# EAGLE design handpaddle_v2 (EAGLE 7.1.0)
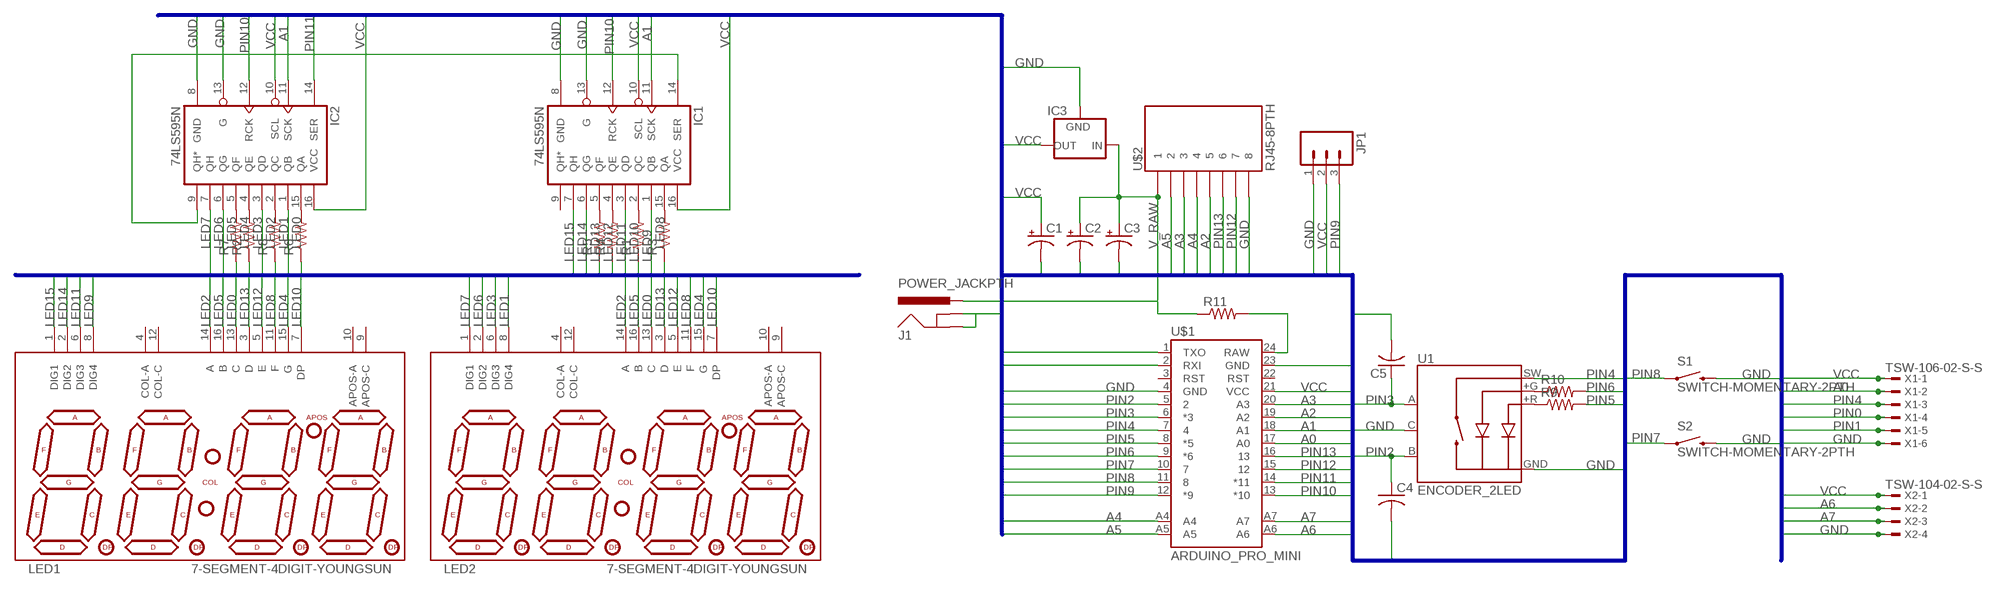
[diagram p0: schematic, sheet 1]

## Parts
C1  CPOL-USE2.5-6  [E2,5-6]
C2  CPOL-USE2.5-6  [E2,5-6]
C3  CPOL-USE2.5-6  [E2,5-6]
C4  C-USC0805  [C0805]
C5  C-USC0805  [C0805]
IC1  74LS595N  [DIL16]
IC2  74LS595N  [DIL16]
IC3  V_REG_78XXSINK  [TO220-IGO]
J1  POWER_JACKPTH  [POWER_JACK_PTH]
JP1  M03PTH  [1X03]
LED1  7-SEGMENT-4DIGIT-YOUNGSUN  [7-SEGMENT-4DIGIT-YOUNGSUN]
LED2  7-SEGMENT-4DIGIT-YOUNGSUN  [7-SEGMENT-4DIGIT-YOUNGSUN]
R1  R-US_R0805  [R0805]
R2  R-US_R0805  [R0805]
R3  R-US_R0805  [R0805]
R4  R-US_R0805  [R0805]
R5  R-US_R0805  [R0805]
R6  R-US_R0805  [R0805]
R7  R-US_R0805  [R0805]
R8  R-US_R0805  [R0805]
R9  R-US_R0805  [R0805]
R10  R-US_R0805  [R0805]
R11  R-US_R0805  [R0805]
S1  SWITCH-MOMENTARY-2PTH  [TACTILE-PTH]
S2  SWITCH-MOMENTARY-2PTH  [TACTILE-PTH]
U1  ENCODER_2LED  [ENCODER_LED_2]
U$1  ARDUINO_PRO_MINI  [ARDUINO_PRO_MINI]
U$2  RJ45-8PTH  [RJ45-8]
X1  TSW-106-02-S-S  [TSW-106-02-S-S]
X2  TSW-104-02-S-S  [TSW-104-02-S-S]

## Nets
A0: U$1.17(A0) X1.2
A1: IC1.11(SCK) IC2.11(SCK) U$1.18(A1)
A2: U$1.19(A2) U$2.5
A3: U$1.20(A3) U$2.3
A4: U$1.A4 U$2.4
A5: U$1.A5 U$2.2
A6: U$1.A6 X2.2
A7: U$1.A7 X2.3
GND: C1.- C2.- C3.- C4.2 C5.2 IC1.8(GND) IC1.13(G) IC2.8(GND) IC2.13(G) IC3.GND J1.GND J1.GNDBREAK JP1.1 S1.3 S2.3 U1.C U1.GND(-) U$1.4(GND) U$1.23(GND) U$2.8 X1.6 X2.4
LED0: LED1.13(C) LED2.13(C) R6.1
LED1: IC2.1(QB) LED2.8(DIG4)
LED2: LED1.14(A) LED2.14(A) R8.1
LED3: IC2.3(QD) LED2.6(DIG3)
LED4: LED1.15(G) LED2.15(G) R2.1
LED5: LED1.16(B) LED2.16(B) R7.1
LED6: IC2.6(QG) LED2.2(DIG2)
LED7: IC2.7(QH) LED2.1(DIG1)
LED8: LED1.11(F) LED2.11(F) R3.1
LED9: IC1.1(QB) LED1.8(DIG4)
LED10: LED1.7(DP) LED2.7(DP) R1.1
LED11: IC1.3(QD) LED1.6(DIG3)
LED12: LED1.5(E) LED2.5(E) R4.1
LED13: LED1.3(D) LED2.3(D) R5.1
LED14: IC1.6(QG) LED1.2(DIG2)
LED15: IC1.7(QH) LED1.1(DIG1)
N$1: IC1.14(SER) IC2.9(QH*)
N$2: IC2.5(QF) R7.2
N$3: IC2.4(QE) R2.2
N$4: IC2.2(QC) R8.2
N$5: IC2.15(QA) R6.2
N$6: IC1.15(QA) R3.2
N$7: IC1.2(QC) R1.2
N$8: IC1.4(QE) R4.2
N$9: IC1.5(QF) R5.2
N$10: R11.2 U$1.24(RAW)
N$11: R9.1 U1.+R
N$12: R10.1 U1.+G
PIN0: U$1.1(TXO) X1.4
PIN1: U$1.2(RXI) X1.5
PIN2: C4.1 U1.B U$1.5
PIN3: C5.1 U1.A U$1.6(*3)
PIN4: U1.SW U$1.7 X1.3
PIN5: R9.2 U$1.8(*5)
PIN6: R10.2 U$1.9(*6)
PIN7: S2.1 U$1.10
PIN8: S1.1 U$1.11
PIN9: JP1.3 U$1.12(*9)
PIN10: IC1.12(RCK) IC2.12(RCK) U$1.13(*10)
PIN11: IC2.14(SER) U$1.14(*11)
PIN12: U$1.15 U$2.7
PIN13: U$1.16 U$2.6
V_RAW: C2.+ C3.+ IC3.IN J1.PWR R11.1 U$2.1
VCC: C1.+ IC1.10(SCL) IC1.16(VCC) IC2.10(SCL) IC2.16(VCC) IC3.OUT JP1.2 U$1.21(VCC) X1.1 X2.1
Unconnected: IC1.9(QH*) LED1.4(COL-A) LED1.9(APOS-C) LED1.10(APOS-A) LED1.12(COL-C) LED2.4(COL-A) LED2.9(APOS-C) LED2.10(APOS-A) LED2.12(COL-C) U$1.3(RST) U$1.22(RST)

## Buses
LED[0..15]
PIN[0..13],A[0..7],VCC,GND

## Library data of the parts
C1-C3 = rcl:CPOL-US: POLARIZED CAPACITOR, American symbol
C4 C5 = rcl:C-US: CAPACITOR, American symbol
IC1 IC2 = SparkFun-DigitalIC:74*595: 8-bit SHIFT REGISTER, output latch
IC3 = SparkFun-PowerIC:V_REG_78XX: Voltage Regulator Standard 7805 5V regulator. IGO (Input Ground Output). Spark Fun Electronics SKU : COM-00107
J1 = SparkFun-Connectors:POWER_JACK: Power Jack This is the standard 5.5mm barrel jack for power. The PTH is the most common, proven, reliable, footprint. The Slot footprint only works if the mill layer is transmitted to the PCB fab house so be warned. Mating wall wart : TOL-00298 (and others); PROD_ID: PRT-00119
JP1 = SparkFun-Connectors:M03: Header 3 Standard 3-pin 0.1" header. Use with straight break away headers (SKU : PRT-00116), right angle break away headers (PRT-00553), swiss pins (PRT-00743), machine pins (PRT-00117), and female headers (PRT-00115). Molex polarized connector foot print use with SKU : PRT-08232 with associated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
LED1 LED2 = SparkFun-Displays:7-SEGMENT-4DIGIT-YOUNGSUN: This is a part for the 4-Digit 7-segment LEDs from Young Sun. Different from the Digikey LEDs, all 16 pins are used. The LONGPADS Variant is used for a test jig, but you may like it because there is more pad to solder to. If you are concerned about routing space, the standard works just fine though.
R1-R11 = rcl:R-US_: RESISTOR, American symbol
S1 S2 = SparkFun-Electromechanical:SWITCH-MOMENTARY-2: Various NO switches- pushbuttons, reed, etc
U1 = SparkFun-Electromechanical:ENCODER_2LED: Illuminated Rotary Encoder w/ 2 LEDs
U$1 = SparkFun-Boards:ARDUINO_PRO_MINI
U$2 = SparkFun-Connectors:RJ45-8: RJ45 Jack Simple RJ45, 8-pin connection - connector for common Cat5, Cat5e, and Cat6 Ethernet cables. Footprint not yet proven in production. Connector sku is PRT-00643; Breakout PCB sku is BOB-00716.
X1 = con-samtec:TSW-106-02-S-S: THROUGH-HOLE .025" SQ POST HEADER Source: Samtec TSW.pdf; OC_FARNELL: unknown; OC_NEWARK: unknown
X2 = con-samtec:TSW-104-02-S-S: THROUGH-HOLE .025" SQ POST HEADER Source: Samtec TSW.pdf; OC_FARNELL: unknown; OC_NEWARK: unknown

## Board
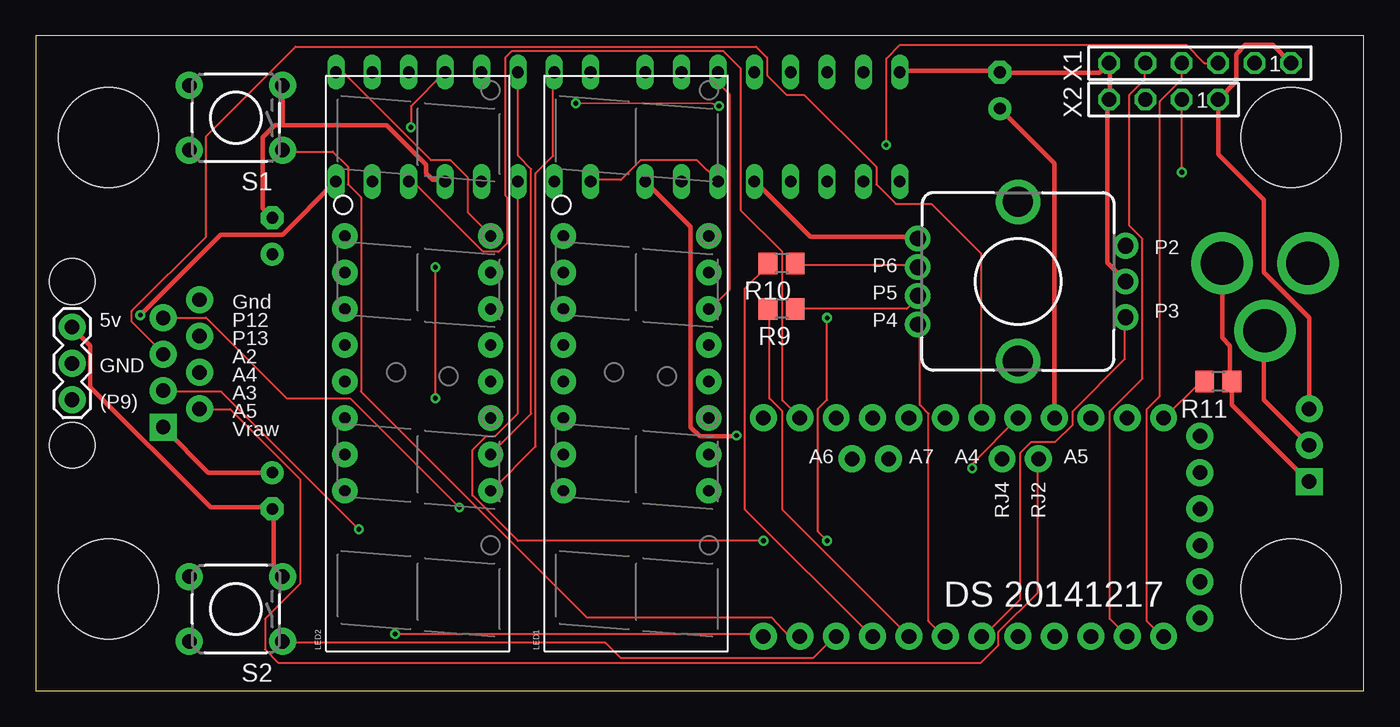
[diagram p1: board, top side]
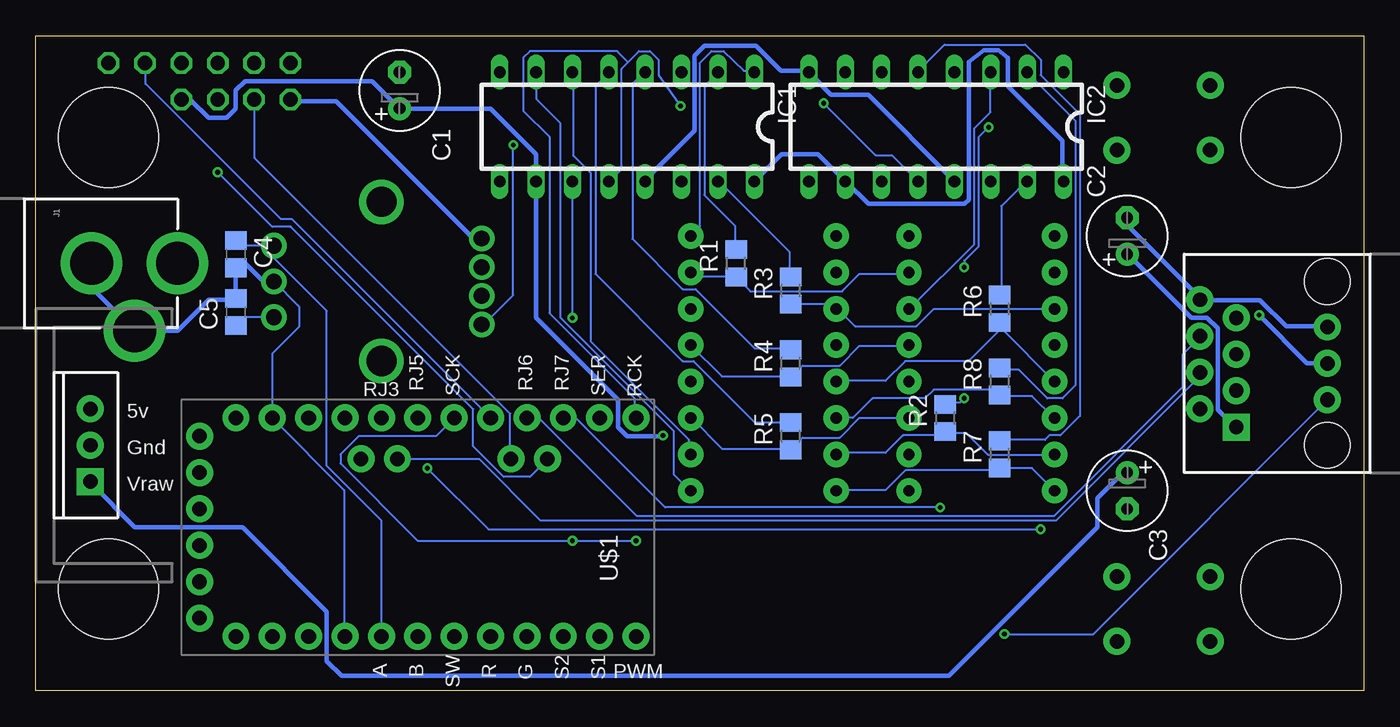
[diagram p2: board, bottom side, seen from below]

Size 92.71 x 45.72 mm. Coordinates in mm from the lower left corner, seen from the top.
Outline: 0,0 92.71,0 92.71,45.72 0,45.72 0,0
Copper layers (1*16): Top 0.0356mm / dielectric 1.5011mm / Bottom 0.0356mm
Design rules "LaenPCBOrder": minimum track width 6mil, minimum drill 13mil, track to track 6mil, track to pad 6mil, pad to pad 6mil, via to via 6mil, smd to smd 6mil, copper to edge 15mil, drill to drill 6mil, minimum pad ring 7mil, minimum via ring 7mil, stop-mask expansion 3mil, vias tented up to drill 0mil, thermal gap 10mil
Holes 6.99 mm at 5.08,38.61 5.08,7.11 87.63,38.61 87.63,7.11

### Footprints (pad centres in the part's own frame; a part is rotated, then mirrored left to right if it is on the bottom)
E2,5-6 = drill 0.813 pad 1.6: + -1.27,0 | drill 0.813 pad 1.6 octagon: - 1.27,0
C0805 = smd 1.3 x 1.5: 1 -0.95,0; 2 0.95,0
DIL16 = drill 0.813 long: 1 -8.89,-3.81; 2 -6.35,-3.81; 3 -3.81,-3.81; 4 -1.27,-3.81; 5 1.27,-3.81; 6 3.81,-3.81; 7 6.35,-3.81; 8 8.89,-3.81; 9 8.89,3.81; 10 6.35,3.81; 11 3.81,3.81; 12 1.27,3.81; 13 -1.27,3.81; 14 -3.81,3.81; 15 -6.35,3.81; 16 -8.89,3.81
TO220-IGO = drill 1 pad 1.88: GND 0,0; OUT 2.54,0 | drill 1 pad 1.88 square: IN -2.54,0
POWER_JACK_PTH = drill 2.997 pad 4.318: GND 0,7.7; GNDBREAK 4.7,10.7; PWR 0,13.7
1X03 = drill 1.016 pad 1.88: 1 0,0; 2 2.54,0; 3 5.08,0
7-SEGMENT-4DIGIT-YOUNGSUN = drill 0.8 pad 1.778: 1 -8.89,-5.08; 2 -6.35,-5.08; 3 -3.81,-5.08; 4 -1.27,-5.08; 5 1.27,-5.08; 6 3.81,-5.08; 7 6.35,-5.08; 8 8.89,-5.08; 9 8.89,5.08; 10 6.35,5.08; 11 3.81,5.08; 12 1.27,5.08; 13 -1.27,5.08; 14 -3.81,5.08; 15 -6.35,5.08; 16 -8.89,5.08
R0805 = smd 1.3 x 1.5: 1 -0.95,0; 2 0.95,0
TACTILE-PTH = drill 1.016 pad 1.88: 1 -3.251,2.261; 2 3.251,2.261; 3 -3.251,-2.261; 4 3.251,-2.261
ENCODER_LED_2 = drill 1.1 pad 1.778: +G 1,7; +R -1,7; GND 3,7; SW -3,7 | drill 1.1 pad 1.8: A -2.5,-7.5; B 2.5,-7.5; C 0,-7.5 | drill 2.1: P$1 -5.55,0; P$2 5.55,0
ARDUINO_PRO_MINI = drill 1.016 pad 1.88: 1 -7.62,12.7; 2 -7.62,10.16; 3 -7.62,7.62; 4 -7.62,5.08; 5 -7.62,2.54; 6 -7.62,0; 7 -7.62,-2.54; 8 -7.62,-5.08; 9 -7.62,-7.62; 10 -7.62,-10.16; 11 -7.62,-12.7; 12 -7.62,-15.24; 13 7.62,-15.24; 14 7.62,-12.7; 15 7.62,-10.16; 16 7.62,-7.62; 17 7.62,-5.08; 18 7.62,-2.54; 19 7.62,0; 20 7.62,2.54; 21 7.62,5.08; 22 7.62,7.62; 23 7.62,10.16; 24 7.62,12.7; A4 4.763,1.429; A5 4.763,3.969; A6 4.763,-9.049; A7 4.763,-6.509; BLK -6.35,15.24; GND -3.81,15.24; GRN 6.35,15.24; RXI 1.27,15.24; TXO 3.81,15.24; VCC -1.27,15.24
RJ45-8 = drill 1 pad 1.88 square: 1 -4.445,6.35 | drill 1 pad 1.88: 2 -3.175,8.89; 3 -1.905,6.35; 4 -0.635,8.89; 5 0.635,6.35; 6 1.905,8.89; 7 3.175,6.35; 8 4.445,8.89 | hole 3.2: -5.715,0; 5.715,0
TSW-106-02-S-S = drill 1 pad 1.5 octagon: 1 6.35,0; 2 3.81,0; 3 1.27,0; 4 -1.27,0; 5 -3.81,0; 6 -6.35,0
TSW-104-02-S-S = drill 1 pad 1.5 octagon: 1 3.81,0; 2 1.27,0; 3 -1.27,0; 4 -3.81,0

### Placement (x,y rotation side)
C1  67.31,41.91 90 bottom
C2  16.51,31.75 90 bottom
C3  16.51,13.97 270 bottom
C4  78.74,30.48 270 bottom
C5  78.74,26.44 90 bottom
IC1  51.44,39.37 180 bottom
IC2  29.84,39.37 180 bottom
IC3  88.9,17.14 90 bottom
J1  96.52,29.84 270 bottom
JP1  2.54,25.4 270 top
LED1  41.91,22.86 90 top
LED2  26.67,22.86 90 top
R1  43.81,29.84 90 bottom
R2  29.21,19.05 90 bottom
R3  40.01,27.94 90 bottom
R4  40.01,22.86 90 bottom
R5  40.01,17.78 90 bottom
R6  25.4,26.67 90 bottom
R7  25.4,16.51 90 bottom
R8  25.4,21.59 90 bottom
R9  52.07,26.67 180 top
R10  52.07,29.84 180 top
R11  82.55,21.59 180 top
S1  13.97,40.01 180 top
S2  13.97,5.71 180 top
U1  68.58,28.57 90 top
U$1  66.04,11.43 90 bottom
U$2  2.54,22.86 90 bottom
X1  81.28,43.81 0 top
X2  78.74,41.27 0 top

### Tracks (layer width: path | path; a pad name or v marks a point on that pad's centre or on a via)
A0
  Bottom 0.152: U$1.17 74.83,32.92 75.59,32.92 85.04,42.37 85.04,43.74 X1.2
A1  (via drill 0.33)
  Top 0.152: IC2.11 33.66,19.37 32.07,17.78 31.43,17.78 30.48,16.83 30.48,13.65 33.66,10.48 v50.8,10.48 | v55.24,26.04 55.24,20.32 54.61,19.68 54.61,11.11 v55.24,10.48
  Bottom 0.152: v50.8,10.48 v55.24,10.48 66.04,10.48 71.44,15.88 71.44,16.51 70.17,17.78 64.77,17.78 U$1.18 | v55.24,26.04 IC1.11
A2
  Top 0.152: U$1.19 65.99,19.05 65.99,30.53 62.53,33.98 60.05,33.98 58.67,35.36 58.67,36.58 53.65,41.6 52.43,41.6 51.05,42.98 51.05,44.2 50.29,44.96 18.14,44.96 11.89,38.71 11.89,31.7 6.71,26.52 6.71,25.76 8.84,23.62 U$2.5
A3  (via drill 0.33)
  Top 0.152: v22.55,11.28 12.95,20.88 8.99,20.88 U$2.3 | v65.38,15.54 65.38,15.85 U$1.20
  Bottom 0.152: v22.55,11.28 61.11,11.28 v65.38,15.54
A4
  Bottom 0.152: U$2.4 11.43,21.95 21.49,11.89 57.45,11.89 61.72,16.15 67.36,16.15 U$1.A4
A5
  Top 0.152: U$1.A5 69.95,16.15 69.95,6.86 67.21,4.12 67.21,3.2 65.99,1.98 16.92,1.98 16,2.9 16,5.03 18.44,7.47 18.44,14.78 13.56,19.66 11.43,19.66 U$2.2
A6  (via drill 0.33)
  Top 0.152: v80.01,36.2 X2.2
  Bottom 0.152: 80.01,41.3 X2.2 | U$1.A6 57,16.15 58.22,14.94 60.05,14.94 62.18,17.07 62.18,19.66 74.92,32.4 74.93,32.38 76.2,32.38 v80.01,36.2
A7
  Bottom 0.152: X2.3 77.42,41.15 77.42,37.19 59.59,19.36 59.59,16.31 U$1.A7
GND
  Top 0.152: 16.61,12.65 C3.- 16.46,12.8 | 17.22,8.08 S2.3 | 2.59,25.3 JP1.1 | 28.5,35.66 IC2.13 | 50.29,35.51 IC1.13 | 61.57,31.7 U1.GND | 74.98,41.3 X2.4 74.83,41.15 | 60.35,43.28 IC1.8 | 67.21,43.28 C1.- 67.36,43.13 | 76.05,28.65 U1.C | 74.98,43.74 74.98,43.13 X1.6 74.98,43.74
  Top 0.305: 16.61,12.65 16.61,8.69 17.22,8.08 | 17.22,39.47 S1.3 | C2.- 15.85,33.68 15.85,38.65 16.67,39.47 17.22,39.47 | 16.46,12.8 12.19,12.8 3.81,21.18 3.81,24.08 2.59,25.3 | 28.5,35.66 27.71,35.66 27.25,36.12 27.25,36.62 27.23,36.64 27.23,36.73 24.49,39.47 17.22,39.47 | 50.29,35.51 54.1,31.7 61.57,31.7 | 67.21,43.28 60.35,43.28 | 74.83,41.15 74.83,29.87 76.05,28.65 | IC3.GND 85.72,20.32 85.72,25.05 J1.GNDBREAK | 67.36,43.13 74.24,43.13 X1.6 | 74.98,43.13 74.98,41.33 X2.4
  Bottom 0.152: 38.71,43.13 IC2.8 38.86,43.28 | 16.46,32.92 C2.- | 11.43,27.43 U$2.8 11.43,27.28 | 2.59,25.45 JP1.1 | 61.72,31.7 U1.GND | 74.83,41.15 X2.4 | U$1.4 71.17,3.81 71.17,14.02 U$1.23 76.2,23.55 74.3,25.45 74.3,26.79 74.39,26.88 U1.C | 50.14,35.66 IC1.13
  Bottom 0.305: 38.71,43.13 37.19,41.6 34.58,41.6 28.67,35.68 28.65,35.66 IC2.13 | 16.46,32.92 16.46,32.46 11.43,27.43 | 2.59,25.45 5.41,25.45 7.24,27.28 11.43,27.28 | 61.72,31.7 62.28,31.7 71.73,41.15 74.83,41.15 | 38.86,43.28 40.68,43.28 42.43,45.03 46.01,45.03 46.71,44.33 46.71,39.09 50.14,35.66 | U1.C 76.83,28.57 78.11,29.84 78.42,29.84 C4.2 C5.2 78.83,27.3 80.64,27.3 82.81,25.14 J1.GNDBREAK 88.82,28.14 J1.GND
LED0
  Bottom 0.152: 25.3,25.3 25.3,25.6 R6.1 25.3,25.3 | LED2.13 25.3,25.3 | 25.3,25.3 27.58,23.01 32,23.01 33.38,21.64 36.73,21.64 LED1.13
LED1
  Top 0.152: IC2.1 21.03,43.13 21.49,43.13 27.58,37.03 28.96,37.03 30.18,35.81 30.18,33.38 31.7,31.85 LED2.8
LED2
  Bottom 0.152: LED2.14 21.64,19.05 23.16,20.57 25.3,20.57 R8.1 25.45,20.73 25.76,21.03 30.02,21.03 30.63,20.42 34.29,20.42 35.66,19.05 LED1.14
LED3
  Bottom 0.152: IC2.3 26.06,43.13 26.06,40.39 27.19,39.25 27.19,31.18 31.7,26.67 LED2.6
LED4
  Bottom 0.152: LED2.15 21.64,16.46 26.21,16.46 27.74,17.98 29.11,17.98 R2.1 29.26,17.98 29.41,17.83 32.16,17.83 33.38,16.61 36.73,16.61 LED1.15
LED5
  Bottom 0.152: LED2.16 23.16,15.54 25.3,15.54 R7.1 25.45,15.54 25.6,15.39 32,15.39 33.38,14.02 36.73,14.02 LED1.16
LED6
  Top 0.152: LED2.2 34.59,19.36 34.59,36.42 33.68,37.34 33.68,43.13 IC2.6
LED7
  Top 0.152: IC2.7 36.12,43.13 36.12,37.34 34.9,36.12 34.9,17.07 31.85,14.02 LED2.1
LED8
  Bottom 0.152: R3.1 39.93,26.98 37.19,26.98 36.88,26.67 LED1.11 36.73,26.67 35.51,25.45 31.24,25.45 30.02,26.67 LED2.11
LED9
  Bottom 0.152: IC1.1 42.67,43.28 43.28,43.28 44.68,44.65 45.54,44.65 46.33,43.84 46.33,32.46 46.94,31.85 LED1.8
LED10
  Bottom 0.152: LED1.7 46.94,29.11 46.79,28.96 43.89,28.96 R1.1 43.74,28.8 42.82,27.89 36.42,27.89 35.2,29.11 31.85,29.11 LED2.7
LED11
  Top 0.152: IC1.3 47.7,43.13 47.7,42.37 48.46,41.6 48.46,28.04 47.09,26.67 LED1.6
LED12
  Bottom 0.152: LED1.5 44.81,21.95 40.08,21.95 R4.1 39.93,21.95 39.17,22.71 36.58,22.71 35.2,24.08 31.85,24.08 LED2.5
LED13
  Bottom 0.152: LED1.3 46.94,19.05 44.81,16.92 40.08,16.92 R5.1 39.93,16.92 39.17,17.68 36.58,17.68 35.2,19.05 LED2.3
LED14
  Bottom 0.152: IC1.6 55.17,43.13 55.17,37.34 53.95,36.12 53.95,24.38 47.09,17.53 47.09,16.61 LED1.2
LED15
  Bottom 0.152: IC1.7 57.76,43.13 57.76,41.3 56.08,39.62 56.08,26.06 48.16,18.14 48.16,15.09 47.09,14.02 LED1.1
N$1
  Top 0.152: IC2.9 38.86,35.66 40.84,35.66 42.22,37.03 46.18,37.03 47.55,35.66 IC1.14
N$2
  Bottom 0.152: R7.2 25.3,17.53 22.25,17.53 21.95,17.83 21.18,17.83 19.81,19.2 19.81,40.23 22.55,42.98 22.55,44.04 23.62,45.11 29.26,45.11 31.09,43.28 IC2.5
N$3  (via drill 0.33)
  Top 0.152: v27.89,29.57 v27.89,20.42 | v26.19,39.34 26.19,40.82 28.5,43.13 IC2.4
  Bottom 0.152: v27.89,20.42 28.19,20.12 29.11,20.12 R2.2 | v27.89,29.57 27.89,30.02 26.89,31.01 26.89,38.64 v26.19,39.34
N$4
  Bottom 0.152: R8.2 25.3,22.4 24.08,22.4 22.1,20.42 21.03,20.42 20.12,21.34 20.12,39.78 23.47,43.13 IC2.2
N$5
  Bottom 0.152: R6.2 25.3,27.74 25.3,33.83 23.62,35.51 IC2.15
N$6
  Bottom 0.152: R3.2 40.08,28.96 40.08,30.63 44.96,35.51 IC1.15
N$7
  Bottom 0.152: R1.2 43.89,30.94 43.89,32.46 46.02,34.59 46.02,42.22 45.11,43.13 IC1.2
N$8
  Bottom 0.152: R4.2 40.08,23.93 42.52,23.93 46.63,28.04 47.55,28.04 51.05,31.55 51.05,42.37 50.29,43.13 IC1.4
N$9
  Bottom 0.152: R5.2 40.08,18.75 42.52,18.75 46.79,23.01 47.55,23.01 53.65,29.11 53.65,42.22 52.73,43.13 IC1.5
N$10
  Top 0.152: R11.2 81.53,21.49 81.23,21.49 78.79,19.05 U$1.24
N$11
  Top 0.152: R9.1 60.81,26.67 61.57,27.43 U1.+R
N$12
  Top 0.152: R10.1 53.03,29.72 61.57,29.72 U1.+G
PIN0
  Top 0.152: X1.4 80.01,42.67 78.49,41.15 78.49,20.57 77.57,19.66 77.57,4.88 78.64,3.81 U$1.1
PIN1
  Top 0.152: U$1.2 74.98,5.03 74.98,19.51 77.27,21.79 77.27,31.55 76.35,32.46 76.35,41.6 77.42,42.67 77.42,43.74 X1.5
PIN2
  Bottom 0.152: U$1.5 68.58,11.89 72.39,15.7 72.39,26.52 76.05,30.18 76.05,30.94 U1.B 78.39,31.07 C4.1
PIN3
  Top 0.152: U1.A 76.05,26.06 76.05,23.16 72.39,19.51 72.39,18.59 71.17,17.37 69.49,17.37 68.73,16.61 68.73,6.4 66.14,3.81 U$1.6
  Bottom 0.152: U1.A 78.39,26.07 C5.1
PIN4  (via drill 0.33)
  Top 0.152: U1.SW 61.72,25.45 61.72,19.96 62.33,19.36 62.33,4.88 63.4,3.81 U$1.7 | X1.3 81.6,43.81 80.33,45.09 60.33,45.09 59.37,44.13 v59.37,38.1
  Bottom 0.152: v59.37,38.1 59.37,27.62 61.28,25.72 U1.SW
PIN5
  Top 0.152: U$1.8 52.12,12.65 52.12,19.51 51.21,20.42 51.21,26.67 R9.2
PIN6
  Top 0.152: R10.2 51.05,29.72 51.05,29.62 49.53,28.09 49.53,12.65 58.37,3.81 U$1.9
PIN7
  Top 0.152: S2.1 17.22,3.35 39.78,3.35 40.84,2.29 54.25,2.29 55.78,3.81 U$1.10
PIN8
  Top 0.152: U$1.11 52.58,3.81 51.36,5.13 38.46,5.13 22.71,20.88 22.71,34.44 21.79,35.36 21.79,36.58 20.73,37.64 17.22,37.64 S1.1
PIN9  (via drill 0.33)
  Top 0.152: v25.08,3.97 50.8,3.97 U$1.12
  Bottom 0.152: JP1.3 18.89,3.97 v25.08,3.97
PIN10  (via drill 0.33)
  Top 0.152: v37.7,41.01 47.24,41 v47.7,40.82
  Bottom 0.152: v37.7,41.01 34.08,37.4 32.95,37.4 IC2.12 | v47.7,40.82 49.23,42.98 49.23,44.04 49.84,44.65 50.6,44.65 51.36,43.89 | 51.36,43.89 51.82,43.43 51.82,36.42 52.58,35.66 IC1.12 | 51.36,43.89 52.12,44.65 58.22,44.65 58.67,44.2 58.67,40.49 56.84,38.66 56.84,26.36 50.9,20.42 50.9,19.05 U$1.13
PIN11
  Top 0.152: U$1.14 52.12,20.27 52.12,30.63 49.23,33.53 49.23,43.43 48.01,44.65 33.22,44.65 32.77,44.2 32.77,34.59 32.92,34.44 32.92,31.24 32.31,30.63 31.24,30.63 26.36,35.51 26.06,35.51 IC2.14
PIN12  (via drill 0.33)
  Top 0.152: v29.57,12.8 21.95,20.42 17.53,20.42 11.89,26.06 8.99,26.06 U$2.7
  Bottom 0.152: U$1.15 55.02,19.05 48.77,12.8 v29.57,12.8
PIN13
  Bottom 0.152: U$1.16 57.61,19.05 50.75,12.19 21.64,12.19 12.65,21.18 12.65,23.47 11.43,24.69 U$2.6
V_RAW
  Top 0.152: 8.99,18.29 U$2.1 | 83.52,21.49 R11.1 83.36,21.64 | 88.85,14.63 IC3.IN
  Top 0.305: C3.+ 12.04,15.24 8.99,18.29 | 83.52,21.49 83.52,19.96 88.85,14.63 | 83.36,21.64 83.36,24.09 82.83,24.64 J1.PWR
  Bottom 0.152: 16.46,30.48 C2.+ | 8.99,18.44 U$2.1 | 16.61,15.24 C3.+ | 88.85,14.48 IC3.IN
  Bottom 0.305: 16.46,30.48 12.04,26.06 10.94,26.06 10.17,25.3 10.17,19.62 8.99,18.44 | 16.61,15.24 16.61,15.44 18.59,13.46 18.59,11.43 28.96,1.07 71.37,1.07 72.39,2.08 72.39,5.54 78.28,11.43 85.8,11.43 88.85,14.48
VCC  (via drill 0.33)
  Top 0.152: 87.63,43.74 X1.1 | 88.85,19.81 IC3.OUT | 20.88,35.51 IC2.16 | 48.9,17.78 v48.92,17.83
  Top 0.305: v7.3,26.23 12.92,31.85 17.22,31.85 20.88,35.51 | 88.85,19.81 88.9,19.81 88.9,26.04 85.72,29.21 85.72,34.29 82.55,37.47 X2.1 83.82,42.55 83.82,44.45 84.45,45.09 86.36,45.09 X1.1 | 87.63,43.74 87.55,43.74 | U$1.21 71.12,36.83 C1.+ | IC1.16 45.72,32.38 45.72,18.41 46.35,17.78 48.9,17.78
  Bottom 0.152: C1.+ | 36.12,35.51 IC2.10 36.27,35.66
  Bottom 0.305: 36.12,35.51 34.59,33.98 27.87,33.98 27.58,34.28 27.58,43.92 26.51,44.72 25.49,44.72 24.83,44.2 24.83,42.18 21.03,38.39 21.03,35.66 IC2.16 | JP1.2 3.96,22.86 v7.3,26.23 | X2.1 81.92,41.27 80.64,40.01 79.38,40.01 78.74,40.64 78.74,41.91 78.11,42.55 69.22,42.55 C1.+ | C1.+ 60.98,40.65 60.96,40.64 57.78,37.47 IC1.10 57.78,26.04 52.07,20.32 52.07,18.41 51.44,17.78 48.97,17.78 v48.92,17.83 | IC1.16 40.64,37.47 38.1,37.47 IC2.10

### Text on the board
tNames: P2 | P6 | Gnd | P5 | P3 | 5v | P12 | P4 | P13 | A2 | GND | A4 | (P9) | A3 | A5 | Vraw | A6 | A7 | A4 | A5 | RJ4 | RJ2 | DS 20141217
bNames: RCK | SER | RJ7 | RJ6 | SCK | RJ5 | RJ3 | 5v | Gnd | Vraw | S1 | S2 | SW | PWM | G | R | B | A

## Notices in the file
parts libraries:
SparkFun-Boards: Licensing: Creative Commons ShareAlike 4.0 International - https://creativecommons.org/licenses/by-sa/4.0
